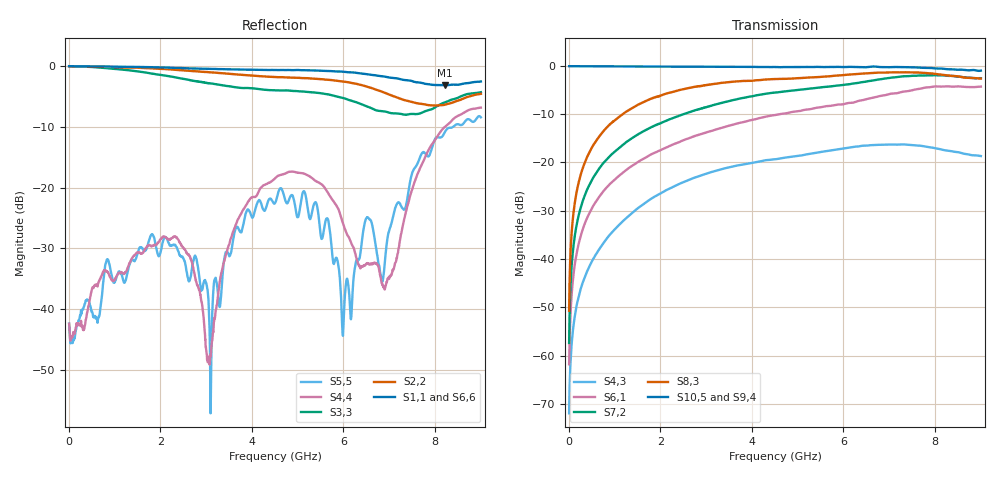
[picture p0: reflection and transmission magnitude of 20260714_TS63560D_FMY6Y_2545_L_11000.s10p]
# GHz S DB R 50
! CMT, SN0916, 25263762, 26.7.0
! Date: 15.07.2026 13:46:48
! Data: Format
! Freq S1.1:dB/Ang S1.2:dB/Ang S1.3:dB/Ang S1.4:dB/Ang S1.5:dB/Ang S1.6:dB/Ang S1.7:dB/Ang S1.8:dB/Ang S1.9:dB/Ang S1.10:dB/Ang
!  S2.1:dB/Ang S2.2:dB/Ang S2.3:dB/Ang S2.4:dB/Ang S2.5:dB/Ang S2.6:dB/Ang S2.7:dB/Ang S2.8:dB/Ang S2.9:dB/Ang S2.10:dB/Ang
!  S3.1:dB/Ang S3.2:dB/Ang S3.3:dB/Ang S3.4:dB/Ang S3.5:dB/Ang S3.6:dB/Ang S3.7:dB/Ang S3.8:dB/Ang S3.9:dB/Ang S3.10:dB/Ang
!  S4.1:dB/Ang S4.2:dB/Ang S4.3:dB/Ang S4.4:dB/Ang S4.5:dB/Ang S4.6:dB/Ang S4.7:dB/Ang S4.8:dB/Ang S4.9:dB/Ang S4.10:dB/Ang
!  S5.1:dB/Ang S5.2:dB/Ang S5.3:dB/Ang S5.4:dB/Ang S5.5:dB/Ang S5.6:dB/Ang S5.7:dB/Ang S5.8:dB/Ang S5.9:dB/Ang S5.10:dB/Ang
!  S6.1:dB/Ang S6.2:dB/Ang S6.3:dB/Ang S6.4:dB/Ang S6.5:dB/Ang S6.6:dB/Ang S6.7:dB/Ang S6.8:dB/Ang S6.9:dB/Ang S6.10:dB/Ang
!  S7.1:dB/Ang S7.2:dB/Ang S7.3:dB/Ang S7.4:dB/Ang S7.5:dB/Ang S7.6:dB/Ang S7.7:dB/Ang S7.8:dB/Ang S7.9:dB/Ang S7.10:dB/Ang
!  S8.1:dB/Ang S8.2:dB/Ang S8.3:dB/Ang S8.4:dB/Ang S8.5:dB/Ang S8.6:dB/Ang S8.7:dB/Ang S8.8:dB/Ang S8.9:dB/Ang S8.10:dB/Ang
!  S9.1:dB/Ang S9.2:dB/Ang S9.3:dB/Ang S9.4:dB/Ang S9.5:dB/Ang S9.6:dB/Ang S9.7:dB/Ang S9.8:dB/Ang S9.9:dB/Ang S9.10:dB/Ang
!  S10.1:dB/Ang S10.2:dB/Ang S10.3:dB/Ang S10.4:dB/Ang S10.5:dB/Ang S10.6:dB/Ang S10.7:dB/Ang S10.8:dB/Ang S10.9:dB/Ang S10.10:dB/Ang
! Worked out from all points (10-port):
!   2001 points, 10 MHz to 9 GHz, reference 50 ohm
!   strongest paths, dB at 10 MHz, 2.257 GHz, 4.505 GHz, 6.753 GHz, 9 GHz:
!     S10,5: -0.1, -0.2, -0.2, -0.2, -1.0
!     S9,4: -0.1, -0.2, -0.4, -0.4, -1.5
!     S8,3: -50.7, -5.4, -2.7, -1.4, -2.6
!     S7,2: -57.4, -10.9, -5.5, -2.8, -2.6
!     S6,1: -61.8, -16.4, -10.2, -6.3, -4.3
!     S4,3: -71.9, -25.2, -19.3, -16.4, -18.7
!   lowest |S11| = -3.2 dB at 8.209 GHz (marker M1), VSWR 5.56, Z = 11.1 - j23.6 ohm
!   |S11| at or under -10 dB: nowhere
